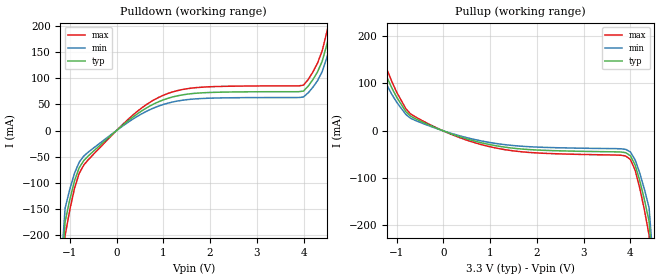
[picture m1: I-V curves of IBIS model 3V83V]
[IBIS Ver]   2.1
[File name]   ics503_3.ibs
[File Rev]   2.0
[Date]   10/24/00
[Source]   ICS MicroClock Applications Engineering 2
[Disclaimer]   This information is for modeling purposes only, and is
|   not guaranteed.
[Component]   ICS503
[Manufacturer] Integrated Circuit Systems Inc.
[Package]
|   typ   min   max
R_pkg   40m   35m   45m
L_pkg   1.65nH   1.35nH   1.95nH
C_pkg   0.24pF   0.14pF   0.34pF
[pin]   signal_name   model_name   R_pin   L_pin   C_pin
   5   CLK   3V83V
| Models and submodels in the file (1): 3V83V (Output)
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|   ICS503 3.3V Clock Drive Model
| This model is suitable for CLK output pins on the
| ICS503
[Model]   3V83V
Model_type   Output
Polarity   Non-Inverting
|   typ   min   max
C_comp   5pF   4pF   6pF
|   typ   min   max
[Voltage range]  3.3V   3.15V   3.45V
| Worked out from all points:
|   slope of the pulldown table from 0 to 0.495 V, typ, clamps not added: 14.2 ohm
|   slope of the pullup table from 0 to 0.495 V, typ, clamps not added: 29.7 ohm
[pulldown]
|Voltage I (typ)   I (min)   I (max)
-3.3V     -3A        -3A        -3A
-1.1V     -174.4mA   -148.3mA   -200.6mA
-900mV    -96.21mA   -81.78mA   -110.6mA
-700mV    -57.29mA   -48.7mA    -65.89mA
300mV     22.3mA     18.95mA    25.64mA
1V        58.6mA     49.81mA    67.39mA
1.8V      71.93mA    61.14mA    82.72mA
4V        75.48mA    64.16mA    86.8mA
4.3V      112.2mA    95.35mA    129mA
4.5V      164.5mA    139.8mA    189.1mA
4.6V      200.2mA    170.1mA    230.2mA
6.6V      3A         3A         3A
[pullup]
|Voltage I (typ)   I (min)   I (max)
-3.3V     3A         3A         3A
-1.4V     193.6mA    164.5mA    222.6mA
-1.2V     110.6mA    94.01mA    127.2mA
-800mV    39.54mA    33.61mA    45.47mA
-200mV    7.146mA    6.074mA    8.218mA
1.4V      -36.23mA   -30.79mA   -41.66mA
3.9V      -46.81mA   -39.79mA   -53.84mA
4V        -53.15mA   -45.18mA   -61.12mA
4.1V      -72.39mA   -61.53mA   -83.25mA
4.2V      -105.5mA   -89.67mA   -121.3mA
4.4V      -191.9mA   -163.1mA   -220.7mA
6.6V      -3A        -3A        -3A
[Ramp]
|   typ   min   max
dV/dt_r   1.38/1.00n   1.31/1.10n   1.46/0.90n
dV/dt_f   1.57/0.9n   1.49/0.99n   1.65/0.81n
